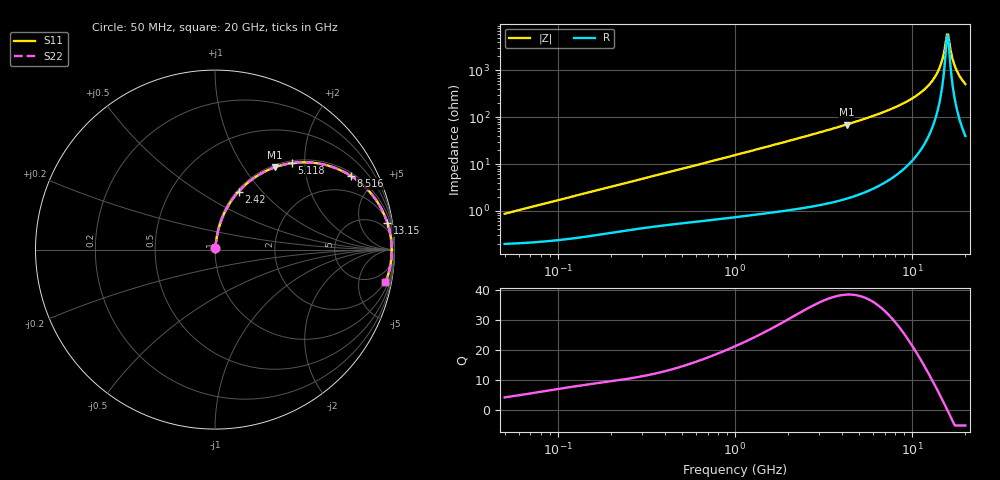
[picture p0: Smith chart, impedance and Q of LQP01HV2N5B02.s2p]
!Murata Part Number: LQP01HV2N5B02
!These Parameters are Measured in Series Mode Connection
!  o--[Z]--o
!Port1  Port2
!  o-------o
!Freq. Start=50[MHz] Stop=20[GHz], 401[Steps]
# Hz S RI R 50
!Freq.(Hz) S11(Real) S11(Imag) S21(Real) S21(Imag) S12(Real) S12(Imag) S22(Real) S22(Imag)
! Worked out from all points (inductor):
!   401 points, 50 MHz to 20 GHz, reference 50 ohm
!   read as one part in series: L = 2.68 nH near 51.52 MHz
!   highest Q = 38.3 at 4.276 GHz (marker M1), where L = 2.6 nH
!   self-resonance near 15.74 GHz
!   S11 on the Smith chart (normalised r, x): 50 MHz: 1.00, +0.02; 2.42 GHz: 1.02, +0.75; 5.118 GHz: 1.05, +1.73; 8.516 GHz: 1.13, +3.62; 13.15 GHz: 2, +13; 20 GHz: 2, -10
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5e7  0.00203 0.00841  0.998 -0.00841  0.998 -0.00841  0.00203 0.00841
1.364002e8  0.00323 0.0225  0.9968 -0.0225  0.9968 -0.0225  0.00323 0.0225
3.721004e8  0.00815 0.0584  0.9919 -0.0584  0.9919 -0.0584  0.00815 0.0584
1e9  0.0301 0.149  0.9699 -0.149  0.9699 -0.149  0.0301 0.149
2.419936e9  0.1317 0.3234  0.8683 -0.3234  0.8683 -0.3234  0.1317 0.3234
2.728004e9  0.1613 0.3537  0.8387 -0.3537  0.8387 -0.3537  0.1613 0.3537
4.275624e9  0.3319 0.458  0.6681 -0.458  0.6681 -0.458  0.3319 0.458
5.117541e9  0.4296 0.482  0.5704 -0.482  0.5704 -0.482  0.4296 0.482
7.442007e9  0.6705 0.4544  0.3295 -0.4544  0.3295 -0.4544  0.6705 0.4544
8.516016e9  0.7579 0.4104  0.2421 -0.4104  0.2421 -0.4104  0.7579 0.4104
1.098561e10  0.8976 0.2761  0.1024 -0.2761  0.1024 -0.2761  0.8976 0.2761
1.314879e10  0.9606 0.1484  0.0394 -0.1484  0.0394 -0.1484  0.9606 0.1484
1.438523e10  0.9777 0.0782  0.0223 -0.0782  0.0223 -0.0782  0.9777 0.0782
1.482269e10  0.9811 0.0543  0.0189 -0.0543  0.0189 -0.0543  0.9811 0.0543
1.550395e10  0.9839 0.0181  0.0161 -0.0181  0.0161 -0.0181  0.9839 0.0181
1.573793e10  0.9843 0.00597  0.0157 -0.00597  0.0157 -0.00597  0.9843 0.00597
1.597544e10  0.9843 -0.00614  0.0157 0.00614  0.0157 0.00614  0.9843 -0.00614
1.621653e10  0.9841 -0.0182  0.0159 0.0182  0.0159 0.0182  0.9841 -0.0182
1.696185e10  0.9815 -0.0545  0.0185 0.0545  0.0185 0.0545  0.9815 -0.0545
1.774144e10  0.9763 -0.0904  0.0237 0.0904  0.0237 0.0904  0.9763 -0.0904
1.88369e10  0.9653 -0.1374  0.0347 0.1374  0.0347 0.1374  0.9653 -0.1374
2e10  0.9497 -0.183  0.0503 0.183  0.0503 0.183  0.9497 -0.183
